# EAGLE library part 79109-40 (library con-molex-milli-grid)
RECEPTACAL
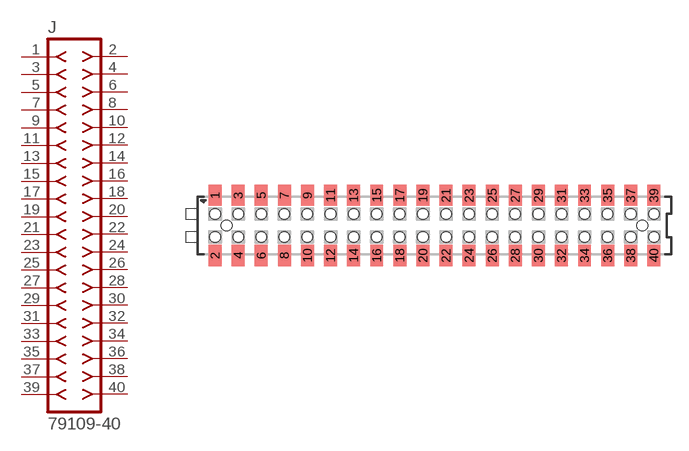
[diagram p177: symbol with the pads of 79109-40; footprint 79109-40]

Designator prefix J

## 79109-40  [79109-40]
1  1  pas
2  2  pas
3  3  pas
4  4  pas
5  5  pas
6  6  pas
7  7  pas
8  8  pas
9  9  pas
10  10  pas
11  11  pas
12  12  pas
13  13  pas
14  14  pas
15  15  pas
16  16  pas
17  17  pas
18  18  pas
19  19  pas
20  20  pas
21  21  pas
22  22  pas
23  23  pas
24  24  pas
25  25  pas
26  26  pas
27  27  pas
28  28  pas
29  29  pas
30  30  pas
31  31  pas
32  32  pas
33  33  pas
34  34  pas
35  35  pas
36  36  pas
37  37  pas
38  38  pas
39  39  pas
40  40  pas

## Footprint 79109-40 (pad centres in mm)
RECEPTACAL SMD Dual Row, Vertical, Pass-Thru
smd 1.12 x 1.83: 1 -19,2.6; 2 -19,-2.6; 3 -17,2.6; 4 -17,-2.6; 5 -15,2.6; 6 -15,-2.6; 7 -13,2.6; 8 -13,-2.6; 9 -11,2.6; 10 -11,-2.6; 11 -9,2.6; 12 -9,-2.6; 13 -7,2.6; 14 -7,-2.6; 15 -5,2.6; 16 -5,-2.6; 17 -3,2.6; 18 -3,-2.6; 19 -1,2.6; 20 -1,-2.6; 21 1,2.6; 22 1,-2.6; 23 3,2.6; 24 3,-2.6; 25 5,2.6; 26 5,-2.6; 27 7,2.6; 28 7,-2.6; 29 9,2.6; 30 9,-2.6; 31 11,2.6; 32 11,-2.6; 33 13,2.6; 34 13,-2.6; 35 15,2.6; 36 15,-2.6; 37 17,2.6; 38 17,-2.6; 39 19,2.6; 40 19,-2.6
hole 0.914 at -18,0
hole 0.914 at -19,1
hole 0.914 at -19,-1
hole 0.914 at -17,-1
hole 0.914 at -17,1
hole 0.914 at -15,-1
hole 0.914 at -15,1
hole 0.914 at 18,0
hole 0.914 at -13,1
hole 0.914 at -13,-1
hole 0.914 at -11,1
hole 0.914 at -11,-1
hole 0.914 at -9,1
hole 0.914 at -9,-1
hole 0.914 at -7,1
hole 0.914 at -7,-1
hole 0.914 at -5,-1
hole 0.914 at -5,1
hole 0.914 at -3,1
hole 0.914 at -3,-1
hole 0.914 at -1,1
hole 0.914 at -1,-1
hole 0.914 at 1,1
hole 0.914 at 1,-1
hole 0.914 at 3,-1
hole 0.914 at 3,1
hole 0.914 at 5,1
hole 0.914 at 7,1
hole 0.914 at 9,1
hole 0.914 at 5,-1
hole 0.914 at 7,-1
hole 0.914 at 9,-1
hole 0.914 at 11,-1
hole 0.914 at 13,-1
hole 0.914 at 15,-1
hole 0.914 at 17,-1
hole 0.914 at 19,-1
hole 0.914 at 11,1
hole 0.914 at 13,1
hole 0.914 at 15,1
hole 0.914 at 17,1
hole 0.914 at 19,1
